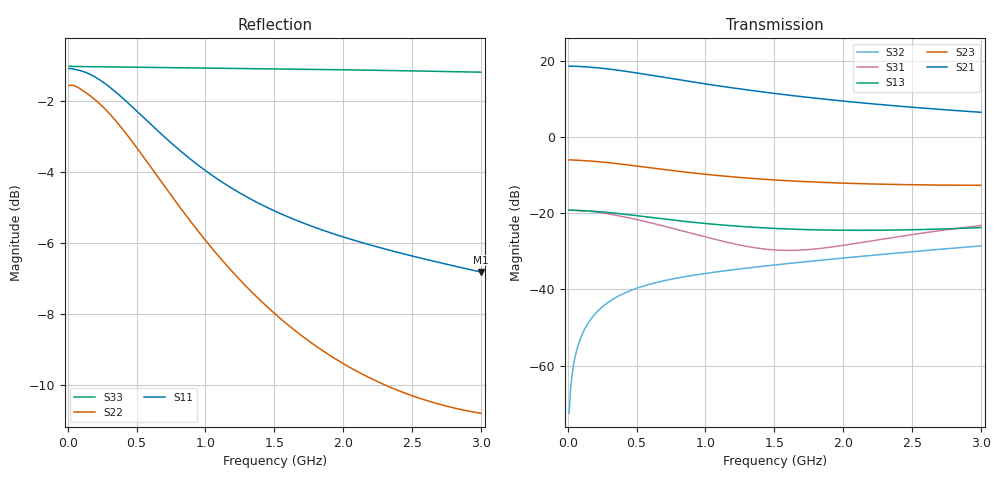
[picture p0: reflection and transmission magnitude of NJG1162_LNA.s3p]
! Created Tue Oct 27 16:08:25 2020
# hz S ma R 50
! 3 Port Network Data from SP1.SP block
! freq  magS11  angS11  magS12  angS12  magS13  angS13
!  magS21  angS21
!  magS22  angS22  magS23  angS23
!  magS31  angS31  magS32  angS32
!  magS33  angS33
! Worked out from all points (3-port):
!   300 points, 10 MHz to 3 GHz, reference 50 ohm
!   strongest paths, dB at 10 MHz, 760 MHz, 1.51 GHz, 2.26 GHz, 3 GHz:
!     S21: 18.7, 15.4, 11.5, 8.6, 6.5
!     S23: -5.9, -8.8, -11.2, -12.3, -12.6
!     S13: -19.1, -21.7, -24.0, -24.4, -23.7
!     S31: -19.1, -23.9, -29.6, -26.9, -23.2
!     S32: -72.5, -37.2, -33.5, -30.9, -28.5
!   lowest |S11| = -6.8 dB at 3 GHz (marker M1), VSWR 2.68, Z = 18.7 - j1.18 ohm
!   |S11| at or under -10 dB: nowhere
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1e7  0.8821 -1.3  0.002105 79.3  0.1106 -0.5
     8.568 179.0  0.8345 -0.9  0.5042 179.2
     0.1105 -0.8  0.0002364 85.4  0.8887 -0.1
8e7  0.8772 -10.5  0.01652 82.4  0.1092 -3.4
     8.506 171.8  0.8282 -8.3  0.4973 173.6
     0.1091 -5.4  0.001965 86.7  0.8876 -0.7
2.8e8  0.8374 -35.7  0.05451 68.8  0.1032 -10.3
       7.93 153.1  0.7704 -26.8  0.4661 160.0
       0.09938 -17.4  0.006514 76.5  0.8868 -2.3
4.1e8  0.7978 -50.6  0.07464 60.6  0.09744 -13.5
       7.389 142.3  0.7199 -37.4  0.4385 152.4
       0.08992 -23.3  0.008927 71.9  0.8862 -3.3
5.4e8  0.7559 -64.0  0.09092 53.6  0.09134 -15.7
       6.808 132.7  0.6663 -46.8  0.4096 146.0
       0.07983 -27.5  0.01095 68.7  0.8855 -4.3
7.6e8  0.6906 -83.6  0.1114 44.2  0.08181 -17.1
       5.873 118.8  0.5815 -60.2  0.3648 137.4
       0.06365 -30.7  0.01374 65.5  0.8843 -6.0
9.8e8  0.6378 -99.9  0.1257 37.1  0.07418 -16.4
       5.08 107.4  0.5111 -70.9  0.3287 130.8
       0.05013 -29.0  0.01605 64.4  0.8832 -7.7
1.51e9  0.555 -129.5  0.1479 25.8  0.06333 -10.0
        3.741 86.2  0.3975 -89.9  0.274 119.8
        0.03302 -2.9  0.02106 65.2  0.8808 -11.8
2.13e9  0.5022 -153.3  0.1668 17.1  0.05986 0.0
        2.832 67.1  0.3283 -104.8  0.2452 110.1
        0.0413 31.5  0.02726 67.6  0.8775 -16.5
3e9  0.4561 -176.9  0.1918 7.1  0.06503 12.1
     2.125 44.5  0.2886 -118.4  0.2334 97.4
     0.06939 41.7  0.03738 69.2  0.8715 -23.3
